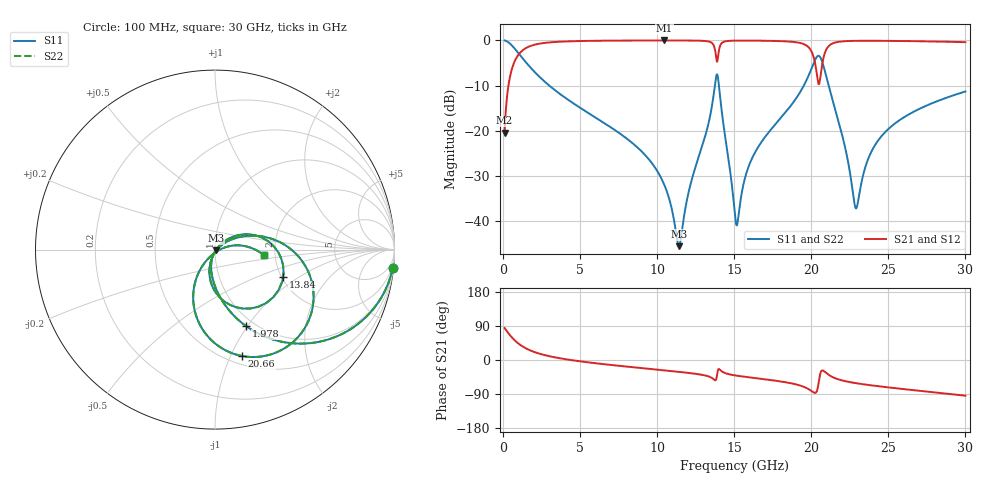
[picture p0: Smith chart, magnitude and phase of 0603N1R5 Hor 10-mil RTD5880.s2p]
# GHz S MA R 50
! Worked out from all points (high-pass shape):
!   3201 points, 100 MHz to 30 GHz, reference 50 ohm
!   highest |S21| = -0.04 dB at 10.45 GHz (marker M1); lowest = -20.4 dB at 100 MHz (marker M2)
!   |S21| within 3 dB of the highest: 1.032 GHz to 13.8 GHz (12.77 GHz wide, 172 % of centre); 20.86 GHz to end of sweep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
!   lowest |S11| = -45.5 dB at 11.42 GHz (marker M3), VSWR 1.01, Z = 50.4 - j0.289 ohm
!   |S11| at or under -10 dB: 2.994 GHz to 13.74 GHz (10.75 GHz wide, 128 % of centre); 14.01 GHz to 19.52 GHz (5.511 GHz wide, 32.9 % of centre); 21.13 GHz to end of sweep
!   |S22| runs from -45.5 to 0.0 dB; largest |S21 - S12| = 0
!   S11 on the Smith chart (normalised r, x): 100 MHz: 1, -20; 1.978 GHz: 0.91, -0.98; 13.84 GHz: 2.04, -0.75; 20.66 GHz: 0.58, -1.11; 30 GHz: 1.74, -0.11
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0.1  0.9954 -5.8  0.09542 84.2  0.09542 84.2  0.9954 -5.8
0.6886562  0.8338 -35.4  0.5516 54.6  0.5516 54.6  0.8338 -35.4
1.978094  0.4594 -68.0  0.8867 21.9  0.8867 21.9  0.4594 -68.0
5.089563  0.1756 -93.1  0.9817 -4.0  0.9817 -4.0  0.1756 -93.1
10.06978  0.03443 -108.5  0.9949 -25.7  0.9949 -25.7  0.03443 -108.5
10.45288  0.0255 -107.0  0.995 -27.3  0.995 -27.3  0.0255 -107.0
11.41528  0.005311 -32.6  0.9945 -31.3  0.9945 -31.3  0.005311 -32.6
13.555  0.1882 26.9  0.9327 -47.5  0.9327 -47.5  0.1882 26.9
13.84466  0.4098 -22.1  0.6154 -48.2  0.6154 -48.2  0.4098 -22.1
14.19037  0.1638 -99.8  0.9317 -29.9  0.9317 -29.9  0.1638 -99.8
15.05  0.01161 -75.3  0.9902 -40.6  0.9902 -40.6  0.01161 -75.3
15.22753  0.009946 -12.9  0.9911 -41.7  0.9911 -41.7  0.009946 -12.9
16.31141  0.05611 34.6  0.9905 -47.5  0.9905 -47.5  0.05611 34.6
18.84356  0.2073 21.9  0.9589 -62.8  0.9589 -62.8  0.2073 21.9
20.03956  0.4995 -8.7  0.7381 -82.6  0.7381 -82.6  0.4995 -8.7
20.34791  0.6514 -36.0  0.4355 -83.2  0.4355 -83.2  0.6514 -36.0
20.65625  0.612 -75.7  0.475 -29.0  0.475 -29.0  0.612 -75.7
21.12344  0.3186 -112.2  0.8605 -38.9  0.8605 -38.9  0.3186 -112.2
22.88941  0.01392 -60.7  0.9858 -61.1  0.9858 -61.1  0.01392 -60.7
23.77706  0.05306 12.0  0.9876 -66.3  0.9876 -66.3  0.05306 12.0
25.01978  0.1053 12.6  0.9849 -72.4  0.9849 -72.4  0.1053 12.6
30  0.2719 -6.0  0.953 -94.2  0.953 -94.2  0.2719 -6.0
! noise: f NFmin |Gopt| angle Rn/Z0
0.1  0.0004568  0.9509  1.096  0.00209
3.417  0.004035  0.81  9.845  0.004394
6.743  0.006835  0.7828  18.84  0.00629
10.06  0.00974  0.7752  27.73  0.008355
13.39  0.02801  0.8902  36.53  0.05009
16.7  0.01701  0.7889  45.19  0.01418
20.03  0.08669  0.9466  53.82  0.2893
23.35  0.02412  0.796  62.18  0.01801
26.67  0.02208  0.7544  70.02  0.0123
30  0.02393  0.7492  77.7  0.01181
